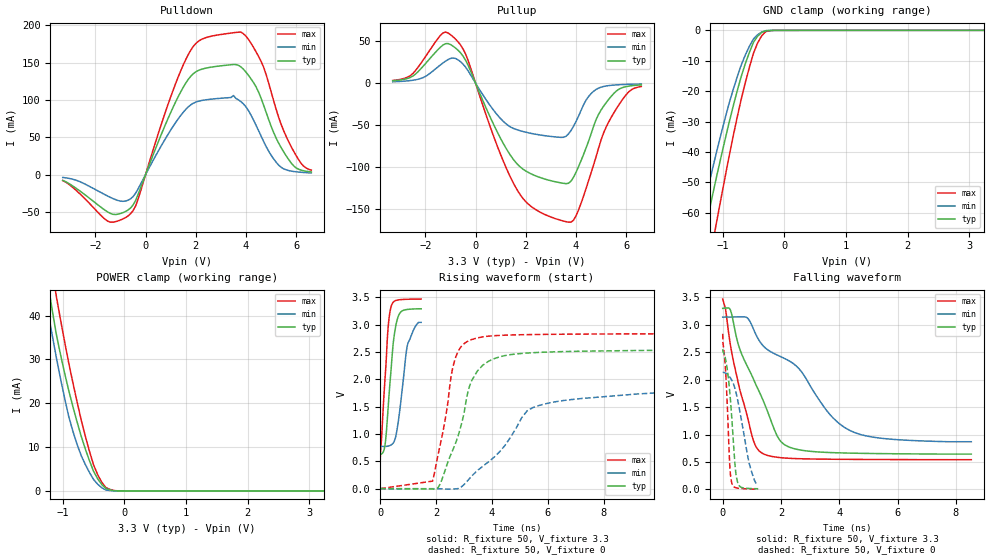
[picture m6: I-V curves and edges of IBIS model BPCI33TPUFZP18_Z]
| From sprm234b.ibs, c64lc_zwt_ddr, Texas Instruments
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[Model]   BPCI33TPUFZP18_Z
Model_type   I/O
Polarity   Non-Inverting
Enable   Active-Low
Vinl =  0.8
Vinh =  2.0
Cref =  10.0000pF
Rref =  50.0000
Vref =  1.5V
Vmeas =  1.5
C_comp   3.402036p   3.350014p   3.525193p
[Temperature Range]   25   125   -40
[Voltage Range]   3.3   3.14   3.47
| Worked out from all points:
|   slope of the pulldown table from 0 to 0.495 V, typ, clamps not added: 11.5 ohm
|   slope of the pullup table from 0 to 0.495 V, typ, clamps not added: 14.2 ohm
|   GND clamp passes 1 mA (typ) near -0.38 V on its own axis
|   POWER clamp passes 1 mA (typ) near -0.33 V on its own axis
|   rising waveform, R_fixture 50, V_fixture 3.3: 20-80 % time 251ps typ, 312ps min, 203ps max; typ from 0.619 V to 3.29 V
|   rising waveform, R_fixture 50, V_fixture 0: 20-80 % time 911ps typ, 3.22ns min, 574ps max; typ from 0 V to 2.55 V
|   falling waveform, R_fixture 50, V_fixture 3.3: 20-80 % time 1.24ns typ, 2.46ns min, 740ps max; typ from 3.3 V to 0.643 V
|   falling waveform, R_fixture 50, V_fixture 0: 20-80 % time 222ps typ, 422ps min, 145ps max; typ from 2.56 V to 0.012 V
[POWER_clamp]
|   voltage   I(typ)   I(min)   I(max)
-3.3V     268.4mA    207.5mA    327.8mA
-1.3V     53.46mA    45.84mA    64.22mA
-1.233V   47.02mA    40.56mA    56.86mA
-1.167V   41.05mA    35.38mA    50.2mA
-1.1V     35.58mA    30.3mA     44.24mA
-900mV    22.84mA    16.94mA    29.12mA
-700mV    12.53mA    8.099mA    16.26mA
-500mV    4.539mA    2.645mA    6.009mA
-366.7mV  1.472mA    729.6uA    2.004mA
-300mV    535.1uA    203.2uA    780.9uA
-100mV    3.165uA    1.607uA    6.874uA
3.233V    -5.948uA   -6.55uA    -6.442uA
[Pulldown]
|   voltage   I(typ)   I(min)   I(max)
-3.3V     -7.786mA   -3.889mA   -7.984mA
-1.5V     -50.3mA    -28.94mA   -62.59mA
-700mV    -47.57mA   -34.42mA   -55.54mA
-400mV    -34.9mA    -25.14mA   -42.3mA
900mV     75.57mA    54.22mA    94.66mA
1.8V      131.8mA    93.47mA    166.8mA
2.4V      142.6mA    100.2mA    183.5mA
3.8V      144.2mA    97.66mA    191mA
4.6V      102.2mA    51.63mA    151.8mA
5.3V      42.12mA    12.63mA    76.7mA
6.1V      7.064mA    3.322mA    19.68mA
6.6V      3.544mA    2.233mA    5.964mA
[Pullup]
|   voltage   I(typ)   I(min)   I(max)
-3.3V     2.841mA    1.735mA    3.327mA
-2.6V     6.941mA    3.146mA    9.055mA
-1.4V     43.04mA    21.88mA    57.16mA
-1V       46.23mA    29.6mA     58.04mA
-400mV    27.63mA    19.3mA     34.95mA
900mV     -60.4mA    -39.07mA   -77.82mA
1.7V      -97.84mA   -56.07mA   -129.6mA
3.7V      -119.6mA   -60.58mA   -166.1mA
4.1V      -99.72mA   -39.32mA   -151.4mA
5.2V      -23.22mA   -3.285mA   -52.37mA
6V        -4.026mA   -1.402mA   -13.56mA
6.6V      -2.032mA   -942.7uA   -3.85mA
[GND_clamp]
|   voltage   I(typ)   I(min)   I(max)
-3.3V     -299.6mA   -234.5mA   -362.2mA
-1.367V   -75.14mA   -63.34mA   -93.5mA
-1.3V     -67.82mA   -57.41mA   -85.56mA
-1.233V   -61.06mA   -51.57mA   -78.06mA
-1.1V     -48.3mA    -40.13mA   -63.31mA
-900mV    -30.76mA   -24.39mA   -41.94mA
-700mV    -15.27mA   -11.5mA    -22.78mA
-500mV    -3.933mA   -2.834mA   -7.527mA
-366.7mV  -681.6uA   -552.6uA   -1.81mA
-300mV    -112.4uA   -122.1uA   -391.1uA
-166.7mV  -11.12uA   -13.5uA    -26.64uA
3.233V    118.1nA    2.958uA    593.5nA
[Ramp]
| variable   typ   min   max
dV/dt_f   1.612353/1.248286n   1.412938/2.563904n   1.764433/0.7425259n
dV/dt_r   1.539412/0.903905n   1.252678/3.797496n   1.706465/0.5751578n
R_load = 50
[Rising Waveform]
R_fixture = 50
V_fixture = 3.3
V_fixture_min = 3.14
V_fixture_max = 3.47
|   time   V(typ)   V(min)   V(max)
0s        618.6mV    772.4mV    535.8mV
8ps       626mV      772.5mV    684.8mV
176ps     820.5mV    772.4mV    2.057V
280ps     1.469V     778.2mV    2.941V
384ps     2.159V     799.1mV    3.322V
488ps     2.762V     854.8mV    3.422V
664ps     3.176V     1.296V     3.453V
984ps     3.278V     2.648V     3.464V
1.264ns   3.288V     2.972V     3.467V
1.464ns   3.29V      3.04V      3.468V
[Rising Waveform]
R_fixture = 50
V_fixture = 0
V_fixture_min = 0
V_fixture_max = 0
|   time   V(typ)   V(min)   V(max)
0s        19.18uV    15.34uV    24.98uV
1.872ns   -6.261mV   -632.7uV   138mV
2.136ns   79.82mV    -1.953mV   778.1mV
2.688ns   822mV      -4.654mV   2.385V
3.2ns     1.88V      187.9mV    2.712V
3.672ns   2.258V     410.4mV    2.777V
4.464ns   2.434V     789.4mV    2.807V
5.256ns   2.48V      1.422V     2.817V
6.648ns   2.508V     1.618V     2.825V
28.78ns   2.554V     2.04V      2.837V
[Falling Waveform]
R_fixture = 50
V_fixture = 3.3
V_fixture_min = 3.14
V_fixture_max = 3.47
|   time   V(typ)   V(min)   V(max)
0s        3.3V       3.14V      3.47V
96ps      3.307V     3.143V     3.296V
264ps     3.269V     3.143V     2.635V
600ps     2.537V     3.146V     1.789V
1.056ns   2.01V      2.922V     886.3mV
1.328ns   1.693V     2.654V     668.3mV
2.096ns   823mV      2.393V     572.8mV
2.616ns   721.7mV    2.201V     559.1mV
4.368ns   660.7mV    1.072V     546.7mV
8.528ns   642.7mV    868.5mV    540.8mV
[Falling Waveform]
R_fixture = 50
V_fixture = 0
V_fixture_min = 0
V_fixture_max = 0
|   time   V(typ)   V(min)   V(max)
0s        2.557V     2.136V     2.837V
8ps       2.509V     2.135V     2.671V
88ps      2.401V     2.122V     2.246V
160ps     2.172V     2.097V     1.501V
240ps     1.786V     2.051V     456.7mV
304ps     1.358V     1.997V     132mV
424ps     434.8mV    1.83V      33.79mV
520ps     115.5mV    1.611V     21.64mV
912ps     16.33mV    469.2mV    7.208mV
1.216ns   11.52mV    101.8mV    3.43mV
